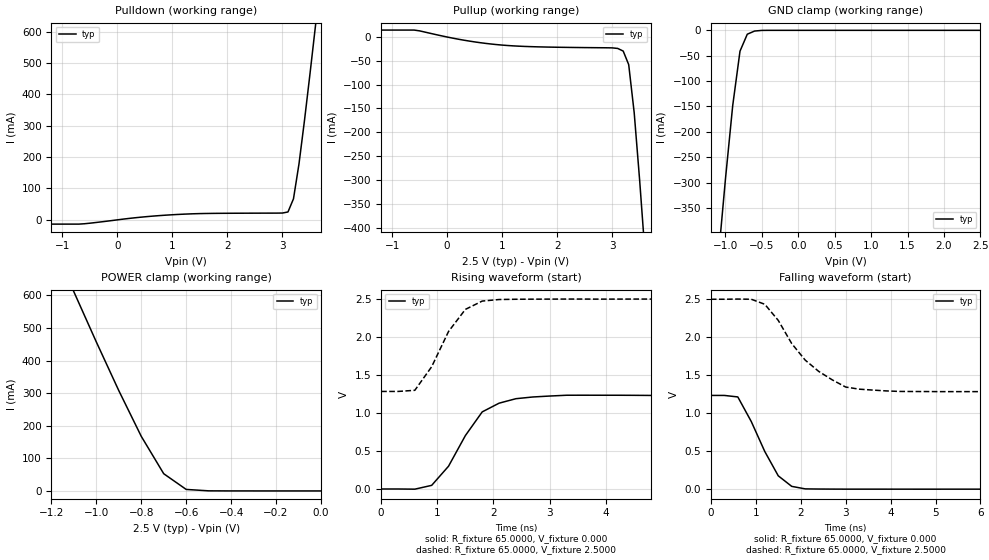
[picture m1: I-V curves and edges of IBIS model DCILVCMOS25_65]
| / 7\'7
| \ \   Xilinx Inc.
| / /
| \_\/.\   IBIS Model for Virtex-II
[IBIS ver]   2.1
[File name]   dci2565.ibs
[File Rev]   1.1
[Date]   Aug. 1, 2001
[Source]   Hspice simulations (08-01: TT, SS, FF)
[Notes]   Xilinx IBIS model for LVDCI 2.5V 65 ohms driver
[Disclaimer] The data in this model is derived from SPICE simulations using
   modeling information extracted from the target process. While
   a great deal of care has been taken to provide information
   that is accurate, this model is considered preliminary as it
   has not been verified by actual silicon measurement. Treat the
   data in this model as preliminary until actual silicon
   verification is performed.
[Copyright]   Copyright 2001, Xilinx Inc., All rights reserved
|   Component Virtex_II
[Component]   Virtex_II
[Manufacturer]   Xilinx Inc.
[Package]
| variable   typ   min   max
R_pkg   0.1000   NA   NA
L_pkg   0.8000nH   NA   NA
C_pkg   0.5000pF   NA   NA
[Pin]  signal_name   model_name   R_pin   L_pin   C_pin
io   DCILVCMOS25_65   DCILVCMOS25_65
| ins  insig   inp
| ens  ensig   inp
PGND   GND   GND
VCCO   VCCO   POWER
| Models and submodels in the file (1): DCILVCMOS25_65 (I/O)
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|   Model DCILVCMOS25_65
[Model]   DCILVCMOS25_65
Model_type   I/O
Polarity   Non-Inverting
Enable   Active-Low
Vinh = 1.7V
Vinl = 0.7V
Vmeas =   1.2000V
Cref =  35.0000pF
Rref =   1.0000M
Vref =  0.000V
C_comp   7.0000pF   NA   NA
[Temperature Range]   25.0000   NA   NA
[Voltage Range]   2.5000V   NA   NA
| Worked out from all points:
|   slope of the pulldown table from 0 to 0.375 V, typ, clamps not added: 49.4 ohm
|   slope of the pullup table from 0 to 0.375 V, typ, clamps not added: 46.8 ohm
|   GND clamp passes 1 mA (typ) near -0.57 V on its own axis
|   POWER clamp passes 1 mA (typ) near -0.52 V on its own axis
|   rising waveform, R_fixture 65.0000, V_fixture 0.000: 20-80 % time 636ps typ, NA min, NA max; typ from 0 V to 1.23 V
|   rising waveform, R_fixture 65.0000, V_fixture 2.5000: 20-80 % time 569ps typ, NA min, NA max; typ from 1.28 V to 2.5 V
|   falling waveform, R_fixture 65.0000, V_fixture 0.000: 20-80 % time 624ps typ, NA min, NA max; typ from 1.23 V to 0 V
|   falling waveform, R_fixture 65.0000, V_fixture 2.5000: 20-80 % time 1.01ns typ, NA min, NA max; typ from 2.5 V to 1.28 V
[Pulldown]
| voltage   I(typ)   I(min)   I(max)
-2.5V     -13.61mA   NA         NA
-700mV    -13.61mA   NA         NA
1V        16.26mA    NA         NA
1.6V      20.28mA    NA         NA
3V        21.72mA    NA         NA
3.1V      25.14mA    NA         NA
3.2V      66.94mA    NA         NA
3.3V      178.1mA    NA         NA
3.4V      316.8mA    NA         NA
3.5V      465.4mA    NA         NA
3.6V      619.1mA    NA         NA
5V        2.882A     NA         NA
[Pullup]
| voltage   I(typ)   I(min)   I(max)
-2.5V     14.58mA    NA         NA
-600mV    14.58mA    NA         NA
300mV     -6.573mA   NA         NA
900mV     -15.91mA   NA         NA
1.5V      -20.13mA   NA         NA
3.1V      -23.96mA   NA         NA
3.2V      -29.52mA   NA         NA
3.3V      -57.95mA   NA         NA
3.4V      -159mA     NA         NA
3.5V      -302.3mA   NA         NA
3.6V      -460.3mA   NA         NA
5V        -2.888A    NA         NA
[GND_clamp]
| voltage   I(typ)   I(min)   I(max)
-2.5V     -2.881A    NA         NA
-1.1V     -452.1mA   NA         NA
-1V       -293.4mA   NA         NA
-900mV    -148.1mA   NA         NA
-800mV    -41.04mA   NA         NA
-700mV    -7.632mA   NA         NA
-600mV    -1.432mA   NA         NA
-500mV    -131.2uA   NA         NA
2.5V      397.5nA    NA         NA
[POWER_clamp]
| voltage   I(typ)   I(min)   I(max)
-2.5V     2.874A     NA         NA
-1.1V     610.9mA    NA         NA
-1V       456.9mA    NA         NA
-900mV    307.7mA    NA         NA
-800mV    167.5mA    NA         NA
-700mV    52.78mA    NA         NA
-600mV    4.607mA    NA         NA
-500mV    279.3uA    NA         NA
0V        397.5nA    NA         NA
[Ramp]
| variable   typ   min   max
dV/dt_r   0.7404/0.6606n   NA   NA
dV/dt_f   0.7296/1.0800n   NA   NA
R_load = 65.0000
[Rising Waveform]
R_fixture = 65.0000
V_fixture = 0.000
| time   V(typ)   V(min)   V(max)
0s        14.09uV    NA         NA
600ps     -2.329mV   NA         NA
900ps     47.87mV    NA         NA
1.2ns     299.6mV    NA         NA
1.5ns     703mV      NA         NA
1.8ns     1.015V     NA         NA
2.1ns     1.129V     NA         NA
2.4ns     1.188V     NA         NA
3.3ns     1.234V     NA         NA
15ns      1.234V     NA         NA
[Rising Waveform]
R_fixture = 65.0000
V_fixture = 2.5000
V_fixture_min = 2.3000
V_fixture_max = 2.7000
| time   V(typ)   V(min)   V(max)
0s        1.284V     NA         NA
300ps     1.284V     NA         NA
600ps     1.299V     NA         NA
900ps     1.609V     NA         NA
1.2ns     2.073V     NA         NA
1.5ns     2.364V     NA         NA
1.8ns     2.474V     NA         NA
2.1ns     2.494V     NA         NA
3ns       2.499V     NA         NA
15ns      2.5V       NA         NA
[Falling Waveform]
R_fixture = 65.0000
V_fixture = 0.000
| time   V(typ)   V(min)   V(max)
0s        1.234V     NA         NA
300ps     1.234V     NA         NA
600ps     1.214V     NA         NA
900ps     889.6mV    NA         NA
1.2ns     495.9mV    NA         NA
1.5ns     175.7mV    NA         NA
1.8ns     36.73mV    NA         NA
2.1ns     3.767mV    NA         NA
15ns      -1.743uV   NA         NA
[Falling Waveform]
R_fixture = 65.0000
V_fixture = 2.5000
V_fixture_min = 2.3000
V_fixture_max = 2.7000
| time   V(typ)   V(min)   V(max)
0s        2.5V       NA         NA
900ps     2.5V       NA         NA
1.2ns     2.434V     NA         NA
1.5ns     2.222V     NA         NA
1.8ns     1.917V     NA         NA
2.1ns     1.698V     NA         NA
2.7ns     1.44V      NA         NA
3ns       1.345V     NA         NA
3.3ns     1.317V     NA         NA
15ns      1.284V     NA         NA
